VAR_GLOBAL CONSTANT	
	// general
	cOversamples			: UDINT := 10;		// number of oversamples
	cSamplerate				: UDINT := 10000;   // 1ms task with 10 oversamples = 10kHz
	cWindowType				: E_CM_WindowType := E_CM_WindowType.eCM_HannWindow;
	cTraceLevel				: TcEventSeverity := TcEventSeverity.Critical;
	
	// define FFT parameters, note that cFSample / cWindowLength must be such that numerical frequency resolution
	// is lower than fLowerFrequencyLimit resolution  =  10000/4000 = 2.5 Hz < 10 Hz 
	cFFTLength				: UDINT	:= 2048;	        // length of FFT
    cWindowLength			: UDINT := 1600;            // 96 samples Zero padding
	cBufferLength			: UDINT	:= cWindowLength/2;	// buffer size due to 50% overlap
	
	// define frequency interval according to ISO 10816-3
	// e.g. 10 .. 1000 Hz for rotating speed over 600r/min
	cMaxBands				: UDINT := 2;
	cfLowerFrequencyLimits	: ARRAY[1..cMaxBands] OF LREAL := [   10,  200];
	cfUpperFrequencyLimits	: ARRAY[1..cMaxBands] OF LREAL := [ 1000, 2000];
	
	// Parameters for RMS calculation
	cOrder       	 		: UDINT := 2; // ISO 10816-3 requires velocity and displacement, if measured using accelerometer we need to integrate 2 times
	cChannels		 		: UDINT := 2; // ISO 10816-3 says 2 orthogonal sensors per measurement location-> 2 channels
	
	// Classes according to ISO: machine type 1, stiff location, Class definitions
	cMemorize				: BOOL := FALSE;
	cMaxClasses				: UDINT := 3;
	cISOClassDef_Vibration	: ARRAY[1..cMaxClasses] OF LREAL := [1E6, 1E6, 1E6];
	cISOClassDef_Velocity	: ARRAY[1..cMaxClasses] OF LREAL := [2.3E-3, 4.5E-3, 7.1E-3];
	cISOClassDef_Displ		: ARRAY[1..cMaxClasses] OF LREAL := [29E-6, 57E-6, 90E-6];	
	
	// optional constants if real sensors are applied
	cGravitationalAcc 		: LREAL := 9.81;    // 1 g approx 9.81 m/s^2 -> physical constant
	cSensitivity      		: LREAL := 0.01;    // [in Volts/g] depends on sensor used in application, e.g. 10 mV/g
	cMeasurementRange 		: LREAL := 5;       // +-5 Volts (EL3632)
	cResolution       		: LREAL := 32768;   // 2^15 (15 bits resolution + 1 bit sign) (EL3632)
	cScale            		: LREAL := cMeasurementRange*cGravitationalAcc/(cSensitivity*cResolution);
END_VAR
